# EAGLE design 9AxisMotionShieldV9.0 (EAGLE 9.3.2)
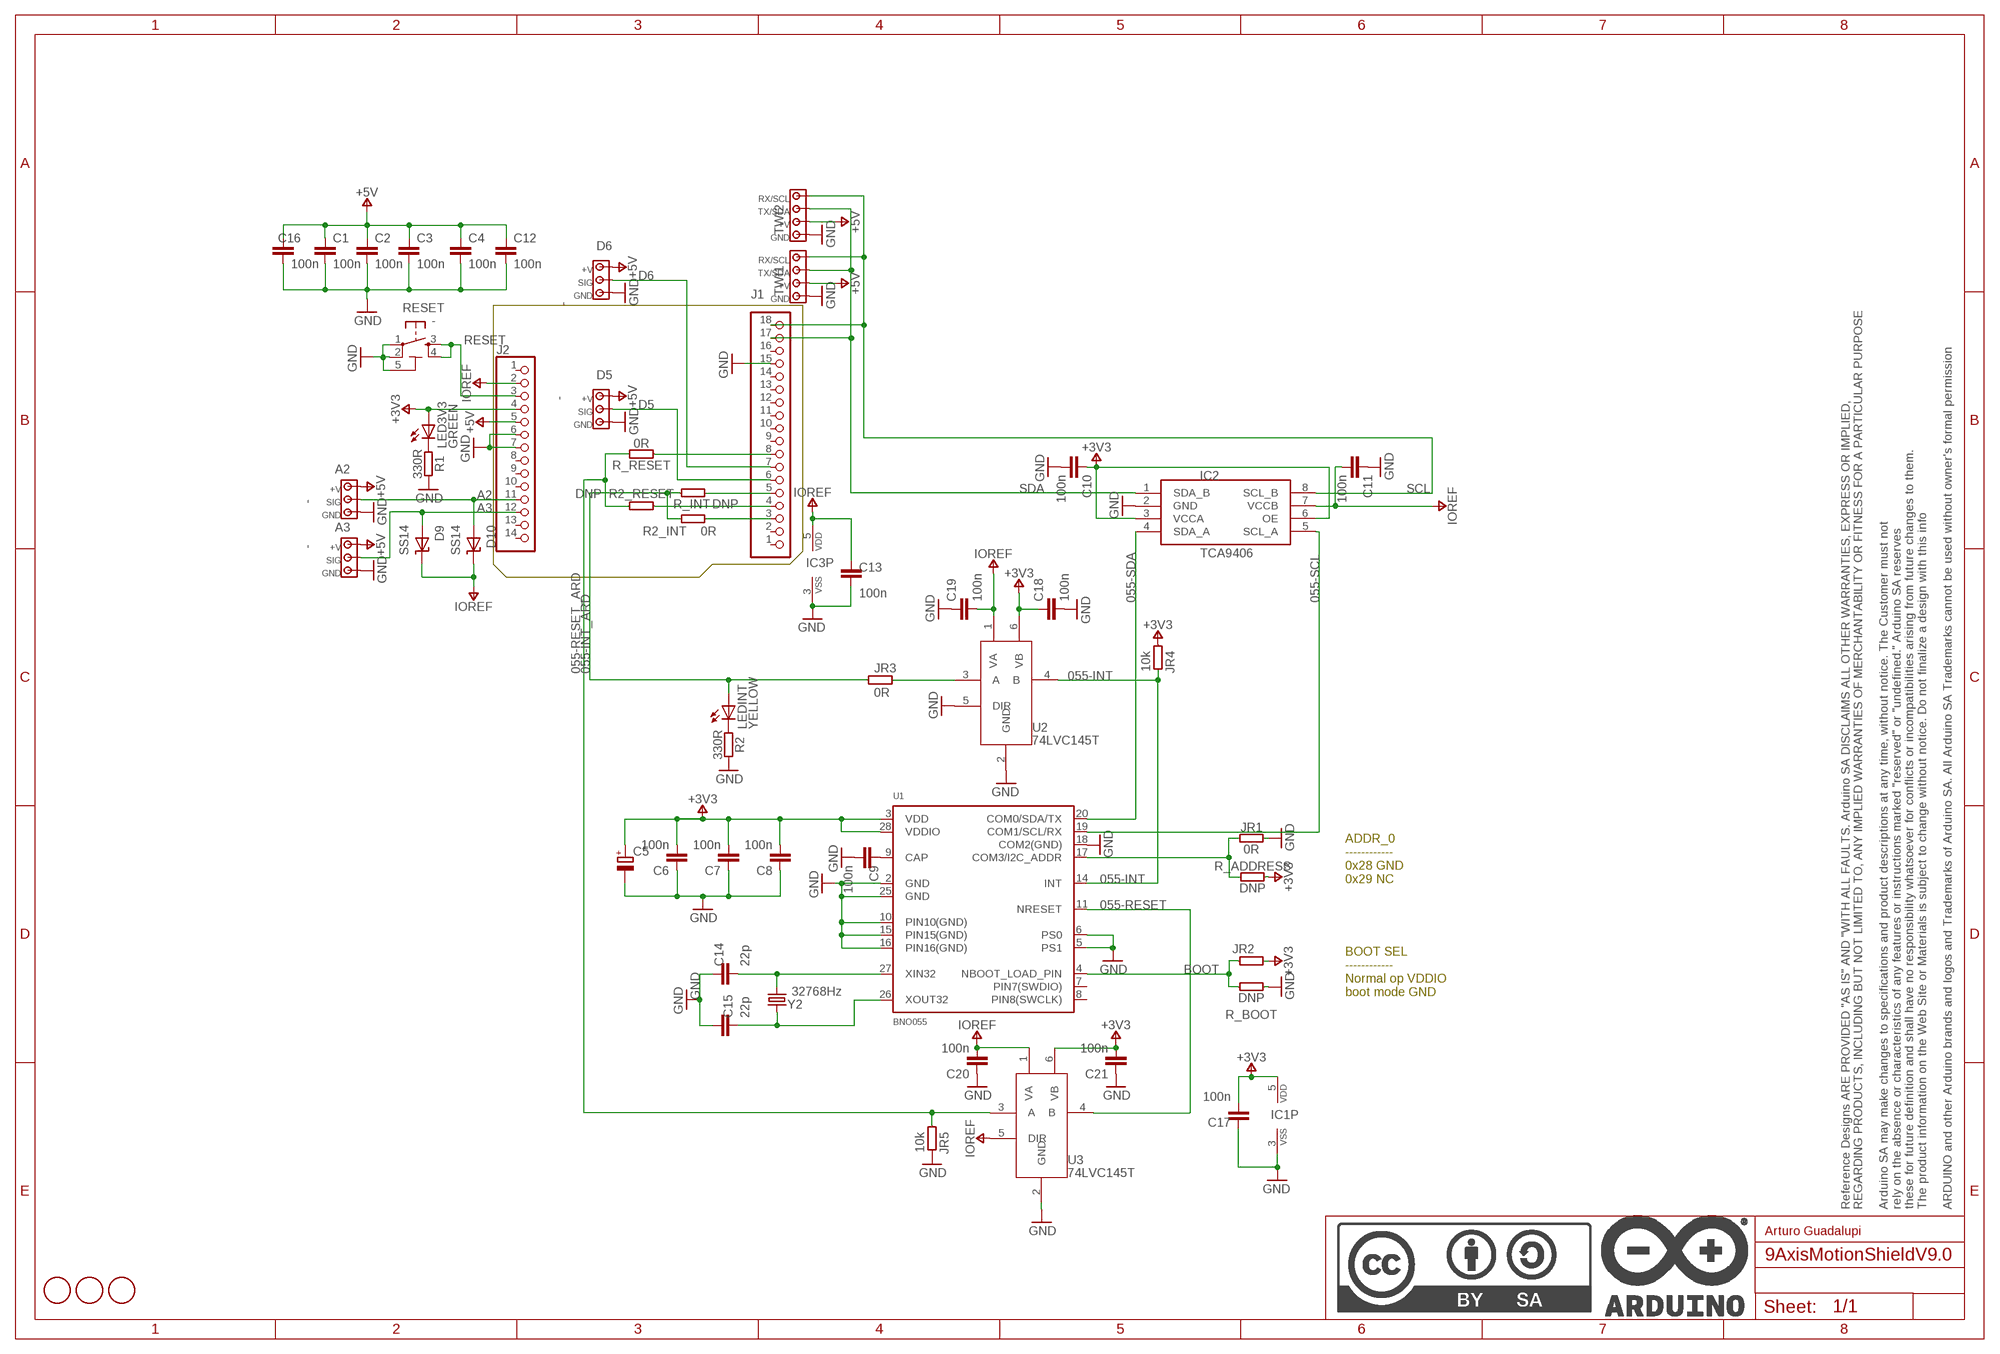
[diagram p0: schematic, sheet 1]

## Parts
A2  -  MODULINO-3  [MODULINO-3]
A3  -  MODULINO-3  [MODULINO-3]
C1  100n  C-100NF-0603  [0603-1608X90N]
C2  100n  C-100NF-0603  [0603-1608X90N]
C3  100n  C-100NF-0603  [0603-1608X90N]
C4  100n  C-100NF-0603  [0603-1608X90N]
C5  22u  0167_  [SMC_B]
C6  100n  C-100NF-0603  [0603-1608X90N]
C7  100n  C-100NF-0603  [0603-1608X90N]
C8  100n  C-100NF-0603  [0603-1608X90N]
C9  100n  C-100NF-0603  [0603-1608X90N]
C10  100n  C-100NF-0603  [0603-1608X90N]
C11  100n  C-100NF-0603  [0603-1608X90N]
C12  100n  C-100NF-0603  [0603-1608X90N]
C13  100n  C-100NF-0603  [0603-1608X90N]
C14  22p  C-22PF-0603  [0603-1608X90N]
C15  22p  C-22PF-0603  [0603-1608X90N]
C16  100n  C-100NF-0603  [0603-1608X90N]
C17  100n  C-100NF-0603  [0603-1608X90N]
C18  100n  C-100NF-0603  [0603-1608X90N]
C19  100n  C-100NF-0603  [0603-1608X90N]
C20  100n  C-100NF-0603  [0603-1608X90N]
C21  100n  C-100NF-0603  [0603-1608X90N]
D5  -  MODULINO-3  [MODULINO-3]
D6  -  MODULINO-3  [MODULINO-3]
D9  SS14  [SMA]
D10  SS14  [SMA]
FID1  DNP  FIDUCIAL-1.5MM  [FD-1-1.5]
FID2  DNP  FIDUCIAL-1.5MM  [FD-1-1.5]
FID3  DNP  FIDUCIAL-1.5MM  [FD-1-1.5]
FRAME1  DNP  A3-FRAME  [FRAME]
IC1  74LVC1G125DCKR  SN74LVC1G125DCKR  [SC70-5]
IC2  TCA9406  [SM-8]
IC3  74LVC1G125DCKR  SN74LVC1G125DCKR  [SC70-5]
J1  PINHD-1X18-SHIELD-CUSTOM  [1X18_]
J2  PINHD-1X14-MALE/FEMALE-CUSTOM  [1X14_]
JR1  0R  R-0R-0402  [0402-1005X55N]
JR2  0R  R-0R-0402  [0402-1005X55N]
JR3  0R  R-0R-0402  [0402-1005X55N]
JR4  10k  R-100K-0603  [C0603]
JR5  10k  R-100K-0603  [C0603]
LED3V3  GREEN  LED-GREEN-0805  [CHIPLED_0805]
LEDINT  YELLOW  LED-YELLOW-0805  [CHIPLED_0805]
R1  330R  R-330R-0402  [0402-1005X55N]
R2  330R  R-330R-0402  [0402-1005X55N]
R2_INT  0R  R-0R-0402  [0402-1005X55N]
R2_RESET  DNP  R-DNP-0402  [0402-1005X55N]
R_ADDRESS  DNP  R-DNP-0402  [0402-1005X55N]
R_BOOT  DNP  R-DNP-0402  [0402-1005X55N]
R_INT  DNP  R-DNP-0402  [0402-1005X55N]
R_RESET  0R  R-0R-0402  [0402-1005X55N]
RESET  -  TACTILE2  [TS42]
TWI1  TWI  MODULINO-4  [MODULINO-4]
TWI2  TWI  MODULINO-4  [MODULINO-4]
U1  BNO055  [BNO055]
U2  74LVC145T  SN74LVC1T45  [DCK]
U3  74LVC145T  SN74LVC1T45  [DCK]
Y2  32768Hz  32.768KHZ  [ABS07]

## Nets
055-INT: JR4.2 U1.14(INT) U2.4(B)
055-INT_ARD: JR3.1 LEDINT.A R2_INT.1 R_INT.1
055-RESET: U1.11(NRESET) U3.4(B)
055-RESET_ARD: JR5.1 R2_RESET.2 R_RESET.2 U3.3(A)
055-SCL: IC2.5(SCL_A) U1.19(COM1/SCL/RX)
055-SDA: IC2.4(SDA_A) U1.20(COM0/SDA/TX)
+3V3 [power]: C5.+ C6.2 C7.2 C8.2 C10.1 C17.2 C18.1 C21.2 IC1.5(VDD) IC2.3(VCCA) IC2.6(OE) J2.4 JR2.2 JR4.1 LED3V3.A R_ADDRESS.2 U1.3(VDD) U1.28(VDDIO) U2.6(VB) U3.6(VB)
+5V [power]: A2.1 A3.1 C1.1 C2.1 C3.1 C4.1 C12.1 C16.1 D5.1 D6.1 J2.5 TWI1.3 TWI2.3
A2: A2.2 D10.P$2(A) J2.11
A3: A3.2 D9.P$2(A) J2.12
ADDR_0: JR1.1 R_ADDRESS.1 U1.17(COM3/I2C_ADDR)
BOOT: JR2.1 R_BOOT.1 U1.4(NBOOT_LOAD_PIN)
D5: D5.2 J1.6
D6: D6.2 J1.7
GND [power]: A2.3 A3.3 C1.2 C2.2 C3.2 C4.2 C5.- C6.1 C7.1 C8.1 C9.2 C10.2 C11.1 C12.2 C13.2 C14.1 C15.1 C16.2 C17.1 C18.2 C19.1 C20.1 C21.1 D5.3 D6.3 IC1.3(VSS) IC2.2(GND) IC3.3(VSS) J1.15 J2.6 J2.7 JR1.2 JR5.2 R1.2 R2.2 R_BOOT.2 RESET.1 RESET.2 RESET.5(5-GND) TWI1.4 TWI2.4 U1.2(GND) U1.5(PS1) U1.6(PS0) U1.10(PIN10(GND)) U1.15(PIN15(GND)) U1.16(PIN16(GND)) U1.18(COM2(GND)) U1.25(GND) U2.2(GND) U2.5(DIR) U3.2(GND)
IOREF: C11.2 C13.1 C19.2 C20.2 D9.P$1(K) D10.P$1(K) IC2.7(VCCB) IC3.5(VDD) J2.2 U2.1(VA) U3.1(VA) U3.5(DIR)
N$1: LED3V3.C R1.1
N$3: C9.1 U1.9(CAP)
N$4: LEDINT.C R2.1
N$7: JR3.2 U2.3(A)
N$8: J1.3 R2_INT.2
N$10: J1.5 R_INT.2
N$11: J1.4 R2_RESET.1
N$56: J1.8 R_RESET.1
RESET: J2.3 RESET.3 RESET.4
SCL: IC2.8(SCL_B) J1.18 TWI1.1 TWI2.1
SDA: IC2.1(SDA_B) J1.17 TWI1.2 TWI2.2
XTAL1: C15.2 U1.26(XOUT32) Y2.1
XTAL2: C14.2 U1.27(XIN32) Y2.2
Unconnected: IC1.1(OE) IC1.2(I) IC1.4(O) IC3.1(OE) IC3.2(I) IC3.4(O) J1.1 J1.2 J1.9 J1.10 J1.11 J1.12 J1.13 J1.14 J1.16 J2.1 J2.8 J2.9 J2.10 J2.13 J2.14 U1.7(PIN7(SWDIO)) U1.8(PIN8(SWCLK))

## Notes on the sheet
- ADDR_0
  ------------
  0x28 GND
  0x29 NC
- BOOT SEL
  ------------
  Normal op VDDIO
  boot mode GND
- Arturo Guadalupi

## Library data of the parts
A2 A3 D5 D6 = Arduino-connectors:MODULINO-3: Polarized lock header 2.54mm pitch; CODE-ARDUINO: A5004; DATASHEET: https://www.alliedelec.com/m/d/412bc68f123f3befd9509afa982df40c.pdf; DISTRIBUTOR-LINK: https://www.alliedelec.com/adam-tech-lha-03-ts/70949176/; DISTRIBUTOR-PN: 70949176; MANUFACTURER: Adam Tech; MANUFACTURER-PN: LHA-03-TS
C1-C4 C6-C13 C16-C21 = Arduino-rcl:C: SMD Capacitor; CODE-ARDUINO: 0015; DATASHEET: http://search.murata.co.jp/Ceramy/image/img/A01X/G101/ENG/GRM188R71C104KA01-01.pdf; DISTRIBUTOR-LINK: https://www.digikey.com/product-detail/en/murata-electronics-north-america/GRM188R71C104KA01D/490-1532-1-ND/587771; DISTRIBUTOR-PN: 490-1532-2-ND; MANUFACTURER: Murata; MANUFACTURER-PN: GRM188R71C104KA01D; NOTE: -; PN-ALTERNATIVE1: NMC0603Y5V104Z25TRPF; PN-ALTERNATIVE2: C1608F104Z500NT; PN-ALTERNATIVE3: C0603C104K3RAC7411; PN-ALTERNATIVE4: 06035D104KAT2A; PN-ALTERNATIVE5: 0603B104K500CT
C5 = Condensatori:0167_: 22uF 25V; MONTHLY_USAGE: _____; PRICE: _____; SUPPLIER: _____; TYPE: Condensatori; VALUE: 22uF
C14 C15 = Arduino-rcl:C: SMD Capacitor; CODE-ARDUINO: 0014; DATASHEET: http://www.samsungsem.com/kr/support/product-search/mlcc/__icsFiles/afieldfile/2016/08/18/S_CL10C220JB8NNNC.pdf; DISTRIBUTOR-LINK: https://www.digikey.com/product-detail/en/samsung-electro-mechanics-america-inc/CL10C220JB8NNNC/1276-1023-1-ND/3889109; DISTRIBUTOR-PN: 1276-1023-1-ND; MANUFACTURER: Samsung; MANUFACTURER-PN: CL10C220JB8NNNC; NOTE: -; PN-ALTERNATIVE1: 0603N220J500CT
D9 D10 = SmartPrj:SS14: DIODE SS14 Diode Schottky 1A 40v
FID1-FID3 = Arduino-utility:FIDUCIAL: Fiducial mount; CODE-ARDUINO: DNP; DATASHEET: DNP; DISTRIBUTOR-LINK: DNP; DISTRIBUTOR-PN: DNP; MANUFACTURER: DNP; MANUFACTURER-PN: DNP
FRAME1 = Arduino-utility:A3-FRAME; CODE-ARDUINO: DNP; DATASHEET: DNP; DISTRIBUTOR-LINK: DNP; DISTRIBUTOR-PN: DNP; MANUFACTURER: DNP; MANUFACTURER-PN: DNP; NOTE: DNP
IC1 IC3 = Arduino-ICs:SN74LVC1G125DCKR: Single bus buffer with 3-state output; CODE-ARDUINO: 0040; DATASHEET: http://www.ti.com/lit/ds/symlink/sn74lvc1g125.pdf; DISTRIBUTOR-LINK: https://www.digikey.com/product-detail/en/texas-instruments/SN74LVC1G125DCKR/296-11604-1-ND/385743; DISTRIBUTOR-PN: 296-11604-1-ND; MANUFACTURER: Texas Instruments; MANUFACTURER-PN: SN74LVC1G125DCKR; NOTE: NO
IC2 = Arduino-ICs:TCA9406: I2C bidirectional level shifter; CODE-ARDUINO: A5381; DATASHEET: http://www.ti.com/lit/ds/symlink/tca9406.pdf; DISTRIBUTOR-LINK: https://www.digikey.com/product-detail/en/texas-instruments/TCA9406DCUR/296-28109-2-ND/2510728; DISTRIBUTOR-PN: 296-28109-2-ND; MANUFACTURER: TI; MANUFACTURER-PN: TCA9406DCUR
J1 = Arduino-connectors:PINHD-1X18: Pin header; CODE-ARDUINO: 3712
J2 = Arduino-connectors:PINHD-1X14: PIN HEADER; CODE-ARDUINO: 3711
JR1-JR3 R2_INT R_RESET = Arduino-rcl:R: SMD Resistor; CODE-ARDUINO: 0039; DATASHEET: www.yageo.com.tw/exep/pages/download/literatures/PYu-R_INT-thick_7.pdf; DISTRIBUTOR-LINK: http://www.digikey.com/product-detail/en/yageo/RC0402FR-070RL/311-0.0LRCT-ND/2827888; DISTRIBUTOR-PN: 311-0.0LRCT-ND; MANUFACTURER: Yageo; MANUFACTURER-PN: RC0402FR-070RL; NOTE: NO
JR4 JR5 = Arduino-rcl:R: SMD Resistor; CODE-ARDUINO: 0026; DATASHEET: http://www.yageo.com/documents/recent/PYu-RC_Group_51_RoHS_L_8.pdf; DISTRIBUTOR-LINK: https://www.digikey.com/product-detail/en/yageo/RC0603FR-07100KL/311-100KHRCT-ND/729836; DISTRIBUTOR-PN: 311-100KHRCT-ND; MANUFACTURER: Yageo; MANUFACTURER-PN: RC0603FR-07100KL; NOTE: NO
LED3V3 = Arduino-diodes:LED: LED; CODE-ARDUINO: 0043; DATASHEET: https://media.digikey.com/pdf/Data%20Sheets/Lite-On%20PDFs/LTST-C170GKT.pdf; DISTRIBUTOR-LINK: https://www.digikey.com/product-detail/it/lite-on-inc/LTST-C170GKT/160-1179-1-ND/269251; DISTRIBUTOR-PN: 160-1179-1-ND; MANUFACTURER: Lite-On; MANUFACTURER-PN: LTST-C170GKT; PN-ALTERNATIVE1: KPT-2012SGC
LEDINT = Arduino-diodes:LED: LED; CODE-ARDUINO: 0044; DATASHEET: https://media.digikey.com/pdf/Data%20Sheets/Lite-On%20PDFs/LTST-C170GKT.pdf; DISTRIBUTOR-LINK: https://www.digikey.com/product-detail/it/lite-on-inc/LTST-C170YKT/160-1175-1-ND/269247; DISTRIBUTOR-PN: 160-1175-1-ND; MANUFACTURER: Lite-On; MANUFACTURER-PN: LTST-C170YKT; PN-ALTERNATIVE1: KPT-2012YC
R1 R2 = Arduino-rcl:R: SMD Resistor; CODE-ARDUINO: 2229; DATASHEET: www.yageo.com.tw/exep/pages/download/literatures/PYu-R_INT-thick_7.pdf; DISTRIBUTOR-LINK: http://www.digikey.com/product-detail/en/yageo/RC0402FR-07330RL/311-330LRCT-ND/729541; DISTRIBUTOR-PN: 311-330LRCT-ND; MANUFACTURER: Yageo; MANUFACTURER-PN: RC0402FR-07330RL; NOTE: NO
R2_RESET R_ADDRESS R_BOOT R_INT = Arduino-rcl:R: SMD Resistor; CODE-ARDUINO: DNP; DATASHEET: DNP; DISTRIBUTOR-LINK: DNP; DISTRIBUTOR-PN: DNP; MANUFACTURER: DNP; MANUFACTURER-PN: DNP; NOTE: NO
RESET = Arduino-pushbuttons:TACTILE2: Pushbutton; CODE-ARDUINO: 0946; DATASHEET: http://www.mouser.com/ds/2/418/NG_CD_1571636_C1-122399.pdf; DISTRIBUTOR-LINK: https://www.mouser.it/ProductDetail/TE-Connectivity/1571636-3/?qs=%2fha2pyFaduiys%2fNUBzym%252bcoSb9tuK3Sjuv54qjf0hQ0%3d; DISTRIBUTOR-PN: 506-1571636-3; MANUFACTURER: TE; MANUFACTURER-PN: 1571636-3; PN-ALTERNATIVE1: TS42031-160WWS027260
TWI1 TWI2 = Arduino-connectors:MODULINO-4: Modulino 4 connector; CODE-ARDUINO: A5005; DATASHEET: https://www.tme.eu/en/Document/21cd81e6196d70241c99017ffcf9ebee/LHA-XX-TS.pdf; DISTRIBUTOR-LINK: https://www.tme.eu/en/details/lha-04-ts/raster-signal-connectors-254mm/adam-tech/; DISTRIBUTOR-PN: LHA-04-TS; MANUFACTURER: ADAM TECH; MANUFACTURER-PN: LHA-04-TS
U1 = Arduino-Sensors:BNO055: BNO055 - Motion Co-Processor; CODE-ARDUINO: 1658; DATASHEET: https://ae-bst.resource.bosch.com/media/_tech/media/datasheets/BST_BNO055_DS000_14.pdf; DISTRIBUTOR-LINK: http://www.digikey.com/product-detail/it/bosch-sensortec/BNO055/828-1058-1-ND/6136309; DISTRIBUTOR-PN: 828-1058-1-ND; MANUFACTURER: Bosch Sensortec; MANUFACTURER-PN: BNO055
U2 U3 = Arduino-ICs:SN74LVC1T45: SINGLE-BIT DUAL-SUPPLY BUS TRANSCEIVER WITH CONFIGURABLE VOLTAGE TRANSLATION AND 3-STATE OUTPUTS DIR = L B to A DIR = H (VVCA) A to B; CODE-ARDUINO: A5331; DATASHEET: http://www.ti.com/lit/ds/symlink/sn74lvc1t45-ep.pdf; DISTRIBUTOR-LINK: https://www.digikey.com/product-detail/en/texas-instruments/SN74LVC1T45DCKR/296-16844-1-ND/639460; DISTRIBUTOR-PN: 296-16844-1-ND; MANUFACTURER: TI; MANUFACTURER-PN: SN74LVC1T45DCKR; NOTE: NO
Y2 = Arduino-crystals:32.768KHZ: LF crystal; CODE-ARDUINO: 0213; DATASHEET: http://www.abracon.com/Resonators/ABS07.pdf; DISTRIBUTOR-LINK: http://www.digikey.com/product-detail/en/abracon-llc/ABS07-32.768KHZ-T/535-9542-1-ND/1237009; DISTRIBUTOR-PN: 535-9542-1-ND; MANUFACTURER: Abracon LLC; MANUFACTURER-PN: ABS07-32.768KHZ-T

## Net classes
1 power: width 0.254 mm, drill 0.3 mm, clearance 0.203 mm

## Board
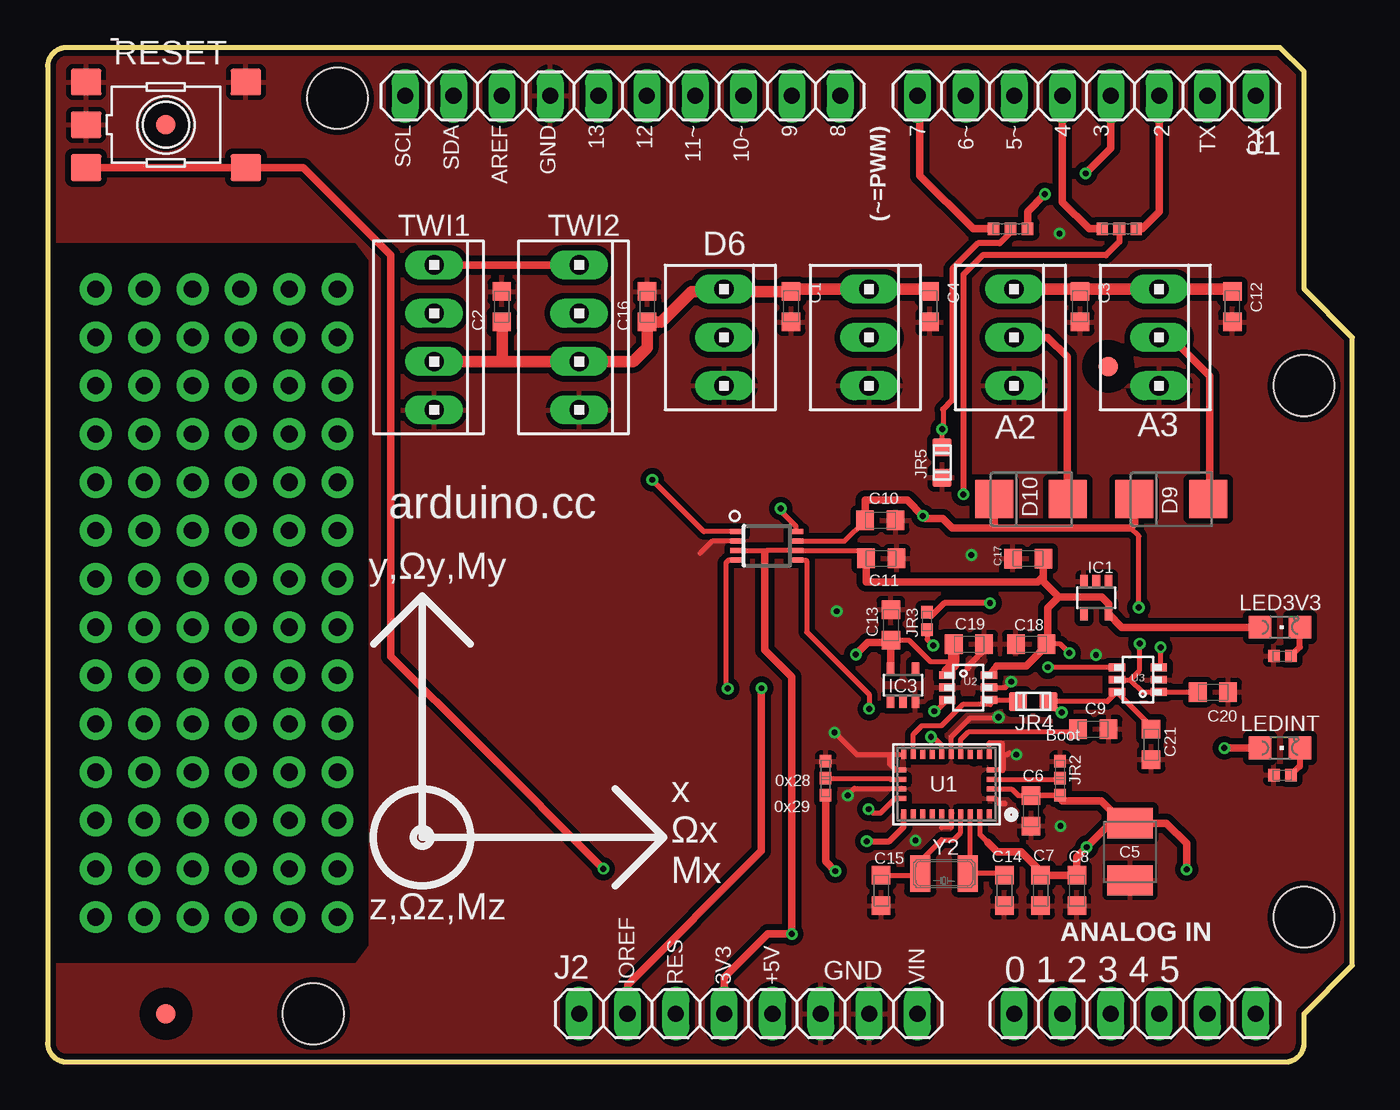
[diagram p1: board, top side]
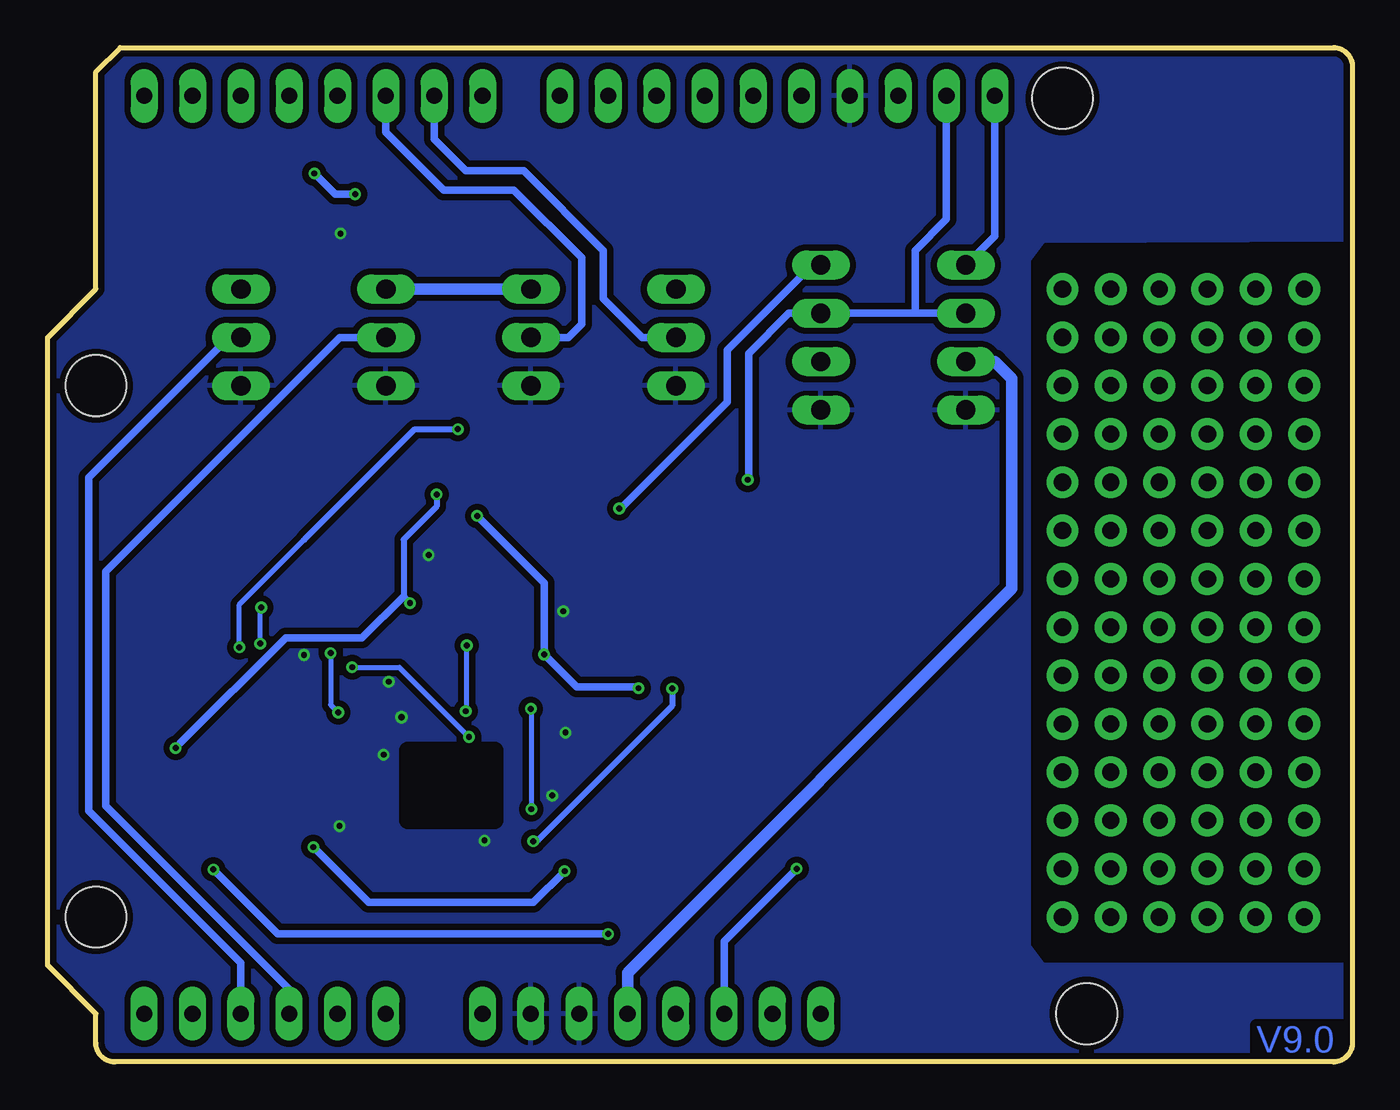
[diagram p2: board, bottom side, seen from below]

Size 68.58 x 53.34 mm. Coordinates in mm from the lower left corner, seen from the top.
Outline: 66.04,2.54 68.58,5.08 68.58,38.1 66.04,40.64 66.04,52.07 64.77,53.34 1,53.34 arc90 0,52.34 0,1 arc90 1,0 65.04,0 arc90 66.04,1 66.04,2.54
Copper layers (1*16): Top 0.035mm / dielectric 1.5mm / Bottom 0.035mm
Design rules "SeeedStudio_2layers *": minimum track width 6mil, minimum drill 0.3mm, track to track 6mil, track to pad 6mil, pad to pad 6mil, via to via 6mil, smd to smd 0mil, copper to edge 10mil, drill to drill 10mil, minimum pad ring 10mil, minimum via ring 6mil, stop-mask expansion 2mil, vias tented up to drill 100mil, thermal gap 10mil
Holes 3.2 mm at 66.04,35.56 66.04,7.62 15.24,50.67 13.97,2.54
tRestrict: 3 lines
bRestrict: 4 lines

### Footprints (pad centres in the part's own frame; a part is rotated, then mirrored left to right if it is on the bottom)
MODULINO-3 = drill 1.016 long: 1 -2.54,0; 2 0,0; 3 2.54,0
0603-1608X90N = smd 0.95 x 1: 1 -0.8,0; 2 0.8,0
SMC_B = smd 1.6 x 2.4: + -1.5,0; - 1.5,0
SMA = smd 2 x 2: P$1 -1.94,0; P$2 1.94,0
FD-1-1.5 = smd 1.016 x 1.016: P$1 0,0
SC70-5 = smd 0.4 x 0.7: 1 -0.65,-0.85; 2 0,-0.85; 3 0.65,-0.85; 4 0.65,0.85; 5 -0.65,0.85
SM-8 = smd 0.25 x 0.75: 1 -0.75,-1.55; 2 -0.25,-1.55; 3 0.25,-1.55; 4 0.75,-1.55; 5 0.75,1.55; 6 0.25,1.55; 7 -0.25,1.55; 8 -0.75,1.55
1X18_ = drill 0.85 pad 1.422 long: 1 -17.78,0; 2 -15.24,0; 3 -12.7,0; 4 -10.16,0; 5 -7.62,0; 6 -5.08,0; 7 -2.54,0; 8 0,0; 9 4.064,0; 10 6.604,0; 11 9.144,0; 12 11.684,0; 13 14.224,0; 14 16.764,0; 15 19.304,0; 16 21.844,0; 17 24.384,0; 18 26.924,0
1X14_ = drill 0.85 pad 1.422 long: 1 -17.78,0; 2 -15.24,0; 3 -12.7,0; 4 -10.16,0; 5 -7.62,0; 6 -5.08,0; 7 -2.54,0; 8 0,0; 9 5.08,0; 10 7.62,0; 11 10.16,0; 12 12.7,0; 13 15.24,0; 14 17.78,0
0402-1005X55N = smd 0.62 x 0.62: 1 -0.45,0; 2 0.45,0
C0603 = smd 0.95 x 1: 1 -0.8,0; 2 0.8,0
CHIPLED_0805 = smd 1.2 x 1.2: A -1.05,0; C 1.05,0
TS42 = smd 1.6 x 1.4: 1 4.2,-2.25; 2 -4.2,-2.25; 3 4.2,2.25; 4 -4.2,2.25; 5 4.2,0
MODULINO-4 = drill 1.016 long: 1 3.81,0; 2 1.27,0; 3 -1.27,0; 4 -3.81,0
BNO055 = smd 0.25 x 0.475: 1 -2.25,1.562; 6 -2.25,-1.562; 7 -1.75,-1.562; 8 -1.25,-1.562; 9 -0.75,-1.562; 10 -0.25,-1.562; 11 0.25,-1.562; 12 0.75,-1.562; 13 1.25,-1.562; 14 1.75,-1.562; 15 2.25,-1.562; 20 2.25,1.562; 21 1.75,1.562; 22 1.25,1.562; 23 0.75,1.562; 24 0.25,1.562; 25 -0.25,1.562; 26 -0.75,1.562; 27 -1.25,1.562; 28 -1.75,1.562 | smd 0.375 x 0.25: 2 -2.312,0.75; 3 -2.312,0.25; 4 -2.312,-0.25; 5 -2.312,-0.75; 16 2.312,-0.75; 17 2.312,-0.25; 18 2.312,0.25; 19 2.312,0.75
DCK = smd 0.9 x 0.4: 1 -1.1,0.65; 2 -1.1,0; 3 -1.1,-0.65; 4 1.1,-0.65; 5 1.1,0; 6 1.1,0.65
ABS07 = smd 1.1 x 1.9: 1 -1.25,0; 2 1.25,0

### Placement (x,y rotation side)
A2  50.8,38.1 270 top
A3  58.42,38.1 270 top
C1  39.08,39.71 270 top
C2  23.87,39.71 90 top
C3  54.27,39.71 270 top
C4  46.35,39.71 270 top
C5  56.9,11.05 270 top
C6  51.69,13.21 90 top
C7  52.2,9.02 90 top
C8  54.1,9.02 90 top
C9  54.97,17.5 0 top
C10  43.82,26.48 0 top
C11  43.77,28.48 180 top
C12  62.27,39.71 270 top
C13  44.32,22.99 90 top
C14  50.29,9.02 90 top
C15  43.81,9.02 90 top
C16  31.51,39.71 90 top
C17  51.54,26.47 0 top
C18  51.69,21.97 180 top
C19  48.43,21.97 180 top
C20  61.25,19.45 180 top
C21  58,16.7 90 top
D5  43.18,38.1 270 top
D6  35.56,38.1 270 top
D9  59.05,29.59 0 top
D10  51.69,29.59 0 top
FID1  6.22,49.28 180 top
FID2  6.22,2.54 0 top
FID3  55.75,36.58 0 top
FRAME1  0,0 0 top
IC1  55.12,24.41 180 top
IC2  37.8,27.14 270 top
IC3  44.96,19.81 0 top
J1  45.72,50.8 180 top
J2  45.72,2.54 0 top
JR1  40.89,15.37 90 top
JR2  53.21,14.48 270 top
JR3  46.22,23.19 270 top
JR4  51.8,18.95 180 top
JR5  47.02,31.52 270 top
LED3V3  64.77,22.86 0 top
LEDINT  64.77,16.51 0 top
R1  64.9,21.35 180 top
R2  64.9,15.08 180 top
R2_INT  56.77,43.81 0 top
R2_RESET  51.05,43.81 180 top
R_ADDRESS  40.89,14.48 270 top
R_BOOT  53.21,15.37 90 top
R_INT  55.88,43.81 180 top
R_RESET  50.16,43.81 0 top
RESET  6.22,49.28 180 top
TWI1  20.32,38.1 90 top
TWI2  27.94,38.1 90 top
U1  47.24,14.61 180 top
U2  48.39,19.68 0 top
U3  57.3,20.1 180 top
Y2  47.12,9.91 0 top

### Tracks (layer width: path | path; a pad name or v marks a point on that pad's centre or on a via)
055-INT
  Top 0.254: U1.14 45.49,17.22 45.95,17.68 46.98,17.68 48.1,18.8 49.55,18.8 U2.4 50.91,19.04 JR4.2
055-INT_ARD  (via drill 0.3)
  Top 0.254: JR3.1 46.42,23.44
  Top 0.305: R2_INT.1 R_INT.1 56.33,43.12 55.63,42.42 49.15,42.42 48.13,41.4 v48.13,29.84 | v49.53,24.13 47.12,24.13 46.42,23.44
  Top 0.406: v61.85,16.51 LEDINT.A
  Bottom 0.305: 61.59,16.76 v61.85,16.51 | v48.13,29.84 48.13,29.21 49.87,27.47 49.87,24.47 v49.53,24.13
  Bottom 0.406: 61.59,16.76 56.07,22.29 52.06,22.29 49.87,24.47
055-RESET  (via drill 0.3)
  Top 0.254: U1.11 46.99,16.64 46.54,17.09 v46.43,17.09 | U3.4 v52.57,20.75
  Bottom 0.254: v46.43,17.09 50.1,20.75 v52.57,20.75
055-RESET_ARD  (via drill 0.3)
  Top 0.254: U3.3 58.5,20.85 v58.5,21.8 | 47.07,34.31 47.07,33.33 v47.02,33.28 JR5.1
  Top 0.305: R_RESET.2 50.62,43.63 50.04,43.05 48.9,43.05 47.55,41.71 47.55,34.8 47.07,34.31
  Top 0.406: R_RESET.2 R2_RESET.2
  Bottom 0.254: v58.5,21.8 58.5,24.05 55.02,27.52
  Bottom 0.305: v47.02,33.28 49.27,33.28 55.02,27.52 55.12,27.43
055-SCL  (via drill 0.3)
  Top 0.254: v43.18,18.57 43.18,19.33 39.9,22.61 39.9,26.35 39.86,26.39 IC2.5 | v43.16,13.3 43.37,13.08 43.78,13.08 44.55,13.86 U1.19
  Bottom 0.254: v43.18,18.57 43.16,18.54 v43.16,13.3
055-SDA  (via drill 0.3)
  Top 0.254: U1.20 | IC2.4 35.79,26.39 35.65,26.25 35.65,19.73 v35.75,19.63
  Top 0.305: v43.05,11.61 44.25,11.61 44.99,12.35 U1.20
  Bottom 0.305: v35.75,19.63 35.75,18.73 42.88,11.61 v43.05,11.61
+3V3  (via drill 0.3)
  Top 0.254: JR2.2 53.33,13.92 53.33,13.72 | 56.64,12.65 56.44,12.65 | U1.3 50.67,14.36 51.02,14.01 51.27,14.01 C6.2 51.73,14.01 51.75,14.03 | U1.28 48.99,11.97 49.4,11.56 | C21.2 58,17.65 U3.6 55.7,18.95 JR4.1 53.17,18.38 v53.3,18.38 | v53.7,21.5 53.23,21.97 C18.1 | C10.1 42.61,26.89 IC2.6 37.77,26.89 | 37.77,26.89 37.69,26.82 | IC2.3 37.77,26.89
  Top 0.305: 51.75,14.03 JR2.2
  Top 0.406: 53.33,13.72 55.37,13.72 56.33,12.76 | 56.33,12.76 56.44,12.65 | 56.33,12.76 56.07,12.76 v54.61,11.3 54.1,10.79 C8.2 C7.2 52.2,10.03 51.18,11.05 49.91,11.05 49.4,11.56 | v41.4,10.03 40.89,10.54 R_ADDRESS.2 | C10.1 43.02,25.25 52.05,25.25 52.34,25.54 | 56.64,12.65 56.74,12.55 C5.+ 58.8,12.55 59.87,11.48 v59.87,10.12 | 52.34,25.54 C17.2 | U2.6 49.88,20.83 51.44,20.83 52.49,21.88 C18.1 52.66,22.14 52.58,22.23 52.58,23.88 53.15,24.45 | 52.34,25.54 52.34,25.26 53.15,24.45 | LED3V3.A 56.47,22.86 IC1.5 55.77,24.08 55.4,24.45 53.15,24.45 | 37.69,26.82 37.7,26.8 37.7,21.66 39.12,20.25 v39.12,6.73 37.85,6.73 35.56,4.45 J2.4
  Bottom 0.254: v53.7,21.5 53.7,18.78 v53.3,18.38
  Bottom 0.406: v41.4,10.03 43.05,8.38 51.69,8.38 v54.61,11.3 | v39.12,6.73 56.48,6.73 v59.87,10.12
+5V
  Top 0.305: D6.1 35.69,40.51
  Top 0.61: C4.1 46.23,40.64 D5.1 39.2,40.64 C1.1 35.69,40.51 33.86,40.51 32.26,38.91 C16.1 31.51,37.55 30.79,36.83 TWI2.3 23.9,36.83 | C3.1 54.39,40.64 | 54.39,40.64 A3.1 62.14,40.64 C12.1 | A2.1 54.39,40.64 | TWI1.3 23.9,36.83 | C2.1 23.9,38.88 23.9,36.83
  Bottom 0.61: TWI1.3 18.8,36.83 17.91,35.94 17.91,24.89 38.1,4.7 J2.5 | D5.1 A2.1
A2
  Top 0.406: D10.P$2 53.59,29.63 53.59,37.08 52.58,38.1 A2.2
  Bottom 0.406: J2.11 55.88,3.81 65.53,13.46 65.53,25.78 53.21,38.1 A2.2
A3
  Top 0.406: D9.P$2 61.09,29.68 61.09,36.07 59.05,38.1 A3.2
  Bottom 0.406: J2.12 58.42,5.21 66.42,13.21 66.42,30.73 59.05,38.1 A3.2
ADDR_0
  Top 0.254: U1.17 44.3,14.86 44.27,14.89 40.92,14.89 JR1.1 | R_ADDRESS.1 40.93,14.81
  Top 0.305: R_ADDRESS.1 JR1.1
BOOT
  Top 0.254: U1.4 53.15,14.86 R_BOOT.1
  Top 0.406: JR2.1 R_BOOT.1 53.15,14.86
D5
  Bottom 0.406: J1.6 50.8,48.9 47.75,45.85 44.07,45.85 40.51,42.29 40.51,38.79 41.2,38.1 D5.2
D6
  Bottom 0.406: J1.7 48.26,48.51 46.61,46.86 43.56,46.86 39.37,42.67 39.37,40.13 37.34,38.1 D6.2
GND  (via drill 0.3, 0.35)
  Top 0.254: 50.55,16.26 50.46,16.17 50.2,16.17 50.16,16.17 50.16,16.75 50.12,16.8 49.5,16.8 49.49,16.79 U1.6 | 50.2,15.36 U1.5 | 47.49,12.32 U1.25 47.54,13.09 | 47.49,12.32 47.5,12.32 | U1.18 44.89,14.4 42.41,14.4 42.05,14.04 v42.05,14.01 | v41.36,17.32 42.52,16.17 44.2,16.17 | 44.2,16.17 U1.15 | 44.2,16.17 44.26,16.1 44.26,15.67 44.58,15.36 U1.16 | 47.49,12.32 46.99,12.32 | U2.5 50.34,19.68 v50.65,20 | IC2.2 34.94,27.39 34.3,26.75 | U1.10 47.49,17.09 47.54,17.14 48.48,18.09 49.93,18.09 v49.97,18.13
  Top 0.305: U1.2 49.77,13.86 50.04,13.59 50.29,13.59 | 50.2,16.17 50.2,15.36 | C19.1 49.23,21.67 48.39,20.83 48.39,20.7
  Top 0.406: C13.2 44.48,24.03
  other vias: 53.24,12.41 41.48,23.7 48.55,26.66 53.19,43.56 45.62,11.65 50.92,16.16 55.1,21.4
  pour Bottom (isolate 0.33): 68.58,0 0,0 0,5.08 16.26,5.08 17.02,6.1 17.02,42.16 16.26,43.18 0,43.26 0,53.34 68.58,53.34
  pour Top (isolate 0.305): 68.58,53.34 68.58,0 0,0 0,5.08 16.26,5.08 17.02,6.1 17.02,42.16 16.26,43.18 0,43.18 0,53.34
IOREF  (via drill 0.3)
  Top 0.254: U3.5 56.9,20.1 | 56.9,20.1 57.55,19.45 U3.1 C20.2 | 56.9,20.1 57.4,20.6 v57.4,22 | v57.35,23.9 57.35,27.65 56.91,28.09 | C13.1 45.26,22.19 46.4,21.05 47.58,21.05 47.59,21.06 47.63,21.1 | 47.29,20.56 U2.1 | IC2.7 41.88,27.39 C11.2
  Top 0.305: IC3.5 44.32,21.06
  Top 0.405: v37.52,19.66 37.52,11.1 30.48,4.06 | v42.48,21.43 43.12,22.06 44.32,22.06 | 46.52,28.57 47.05,28.57
  Top 0.406: 44.32,21.06 44.32,22.06 C13.1 | 49.76,28.07 56.9,28.07 56.91,28.09 57.15,28.32 57.15,29.56 D9.P$1 | 49.76,28.07 49.75,28.08 D10.P$1 | 49.76,28.07 47.56,28.07 47.05,28.57 | C11.2 42.97,29.54 45.17,29.54 v46,28.71 46.14,28.57 46.52,28.57 | J2.2 30.48,4.06
  Top 0.61: 47.29,20.56 47.59,20.86 47.59,21.06 | C19.2 47.63,21.1
  Bottom 0.254: v57.4,22 57.4,23.85 v57.35,23.9
  Bottom 0.405: v37.52,19.66 37.57,19.71 40.77,19.71 v42.48,21.43 42.48,25.2 v46,28.71
N$1
  Top 0.305: R1.1 65.82,21.82 LED3V3.C
N$3
  Top 0.254: U1.9 47.99,16.95 48.4,17.36 54.02,17.36 C9.1
N$4
  Top 0.305: LEDINT.C 65.82,15.57 65.81,15.53 65.8,15.53 R2.1
N$6  (via drill 0.9 pad 1.68)
  other vias: 2.54,33.02
N$7  (via drill 0.3)
  Top 0.254: U2.3 46.7,18.45 v46.6,18.45 | JR3.2 46.22,22.23 v46.55,21.9
  Bottom 0.254: v46.6,18.45 46.55,18.5 v46.55,21.9
N$8
  Top 0.406: J1.3 58.42,44.7 57.53,43.81 R2_INT.2
N$10
  Top 0.406: J1.5 53.34,45.21 54.74,43.81 R_INT.2
N$11  (via drill 0.3)
  Top 0.406: v52.41,45.63 51.5,44.72 R2_RESET.1 | v54.56,46.72 55.88,48.04 J1.4
  Bottom 0.406: v54.56,46.72 53.47,45.63 v52.41,45.63
N$12  (via drill 0.9 pad 1.68)
  other vias: 5.08,33.02
N$13  (via drill 0.9 pad 1.68)
  other vias: 7.62,33.02
N$14  (via drill 0.9 pad 1.68)
  other vias: 10.16,33.02
N$15  (via drill 0.9 pad 1.68)
  other vias: 12.7,33.02
N$16  (via drill 0.9 pad 1.68)
  other vias: 2.54,25.4
N$17  (via drill 0.9 pad 1.68)
  other vias: 5.08,25.4
N$18  (via drill 0.9 pad 1.68)
  other vias: 7.62,25.4
N$19  (via drill 0.9 pad 1.68)
  other vias: 10.16,25.4
N$20  (via drill 0.9 pad 1.68)
  other vias: 12.7,25.4
N$21  (via drill 0.9 pad 1.68)
  other vias: 12.7,22.86
N$22  (via drill 0.9 pad 1.68)
  other vias: 10.16,22.86
N$23  (via drill 0.9 pad 1.68)
  other vias: 7.62,22.86
N$24  (via drill 0.9 pad 1.68)
  other vias: 5.08,22.86
N$25  (via drill 0.9 pad 1.68)
  other vias: 2.54,22.86
N$26  (via drill 0.9 pad 1.68)
  other vias: 2.54,20.32
N$27  (via drill 0.9 pad 1.68)
  other vias: 5.08,20.32
N$28  (via drill 0.9 pad 1.68)
  other vias: 7.62,20.32
N$29  (via drill 0.9 pad 1.68)
  other vias: 10.16,20.32
N$30  (via drill 0.9 pad 1.68)
  other vias: 12.7,20.32
N$31  (via drill 0.9 pad 1.68)
  other vias: 12.7,17.78
N$32  (via drill 0.9 pad 1.68)
  other vias: 10.16,17.78
N$33  (via drill 0.9 pad 1.68)
  other vias: 7.62,17.78
N$34  (via drill 0.9 pad 1.68)
  other vias: 5.08,17.78
N$35  (via drill 0.9 pad 1.68)
  other vias: 2.54,17.78
N$36  (via drill 0.9 pad 1.68)
  other vias: 2.54,15.24
N$37  (via drill 0.9 pad 1.68)
  other vias: 5.08,15.24
N$38  (via drill 0.9 pad 1.68)
  other vias: 7.62,15.24
N$39  (via drill 0.9 pad 1.68)
  other vias: 10.16,15.24
N$40  (via drill 0.9 pad 1.68)
  other vias: 12.7,15.24
N$41  (via drill 0.9 pad 1.68)
  other vias: 12.7,12.7
N$42  (via drill 0.9 pad 1.68)
  other vias: 10.16,12.7
N$43  (via drill 0.9 pad 1.68)
  other vias: 7.62,12.7
N$44  (via drill 0.9 pad 1.68)
  other vias: 5.08,12.7
N$45  (via drill 0.9 pad 1.68)
  other vias: 2.54,12.7
N$46  (via drill 0.9 pad 1.68)
  other vias: 2.54,10.16
N$47  (via drill 0.9 pad 1.68)
  other vias: 5.08,10.16
N$48  (via drill 0.9 pad 1.68)
  other vias: 7.62,10.16
N$49  (via drill 0.9 pad 1.68)
  other vias: 10.16,10.16
N$50  (via drill 0.9 pad 1.68)
  other vias: 12.7,10.16
N$51  (via drill 0.9 pad 1.68)
  other vias: 12.7,7.62
N$52  (via drill 0.9 pad 1.68)
  other vias: 10.16,7.62
N$53  (via drill 0.9 pad 1.68)
  other vias: 7.62,7.62
N$54  (via drill 0.9 pad 1.68)
  other vias: 5.08,7.62
N$55  (via drill 0.9 pad 1.68)
  other vias: 2.54,7.62
N$56
  Top 0.406: R_RESET.1 48.64,43.81 45.85,46.61 45.85,50.67 J1.8
N$62  (via drill 0.9 pad 1.68)
  other vias: 15.24,7.62
N$63  (via drill 0.9 pad 1.68)
  other vias: 15.24,10.16
N$64  (via drill 0.9 pad 1.68)
  other vias: 15.24,12.7
N$65  (via drill 0.9 pad 1.68)
  other vias: 15.24,15.24
N$66  (via drill 0.9 pad 1.68)
  other vias: 15.24,17.78
N$67  (via drill 0.9 pad 1.68)
  other vias: 15.24,20.32
N$68  (via drill 0.9 pad 1.68)
  other vias: 15.24,27.94
N$69  (via drill 0.9 pad 1.68)
  other vias: 15.24,25.4
N$70  (via drill 0.9 pad 1.68)
  other vias: 15.24,22.86
N$71  (via drill 0.9 pad 1.68)
  other vias: 15.24,30.48
N$72  (via drill 0.9 pad 1.68)
  other vias: 12.7,30.48
N$73  (via drill 0.9 pad 1.68)
  other vias: 10.16,30.48
N$74  (via drill 0.9 pad 1.68)
  other vias: 7.62,30.48
N$75  (via drill 0.9 pad 1.68)
  other vias: 5.08,30.48
N$76  (via drill 0.9 pad 1.68)
  other vias: 2.54,30.48
N$77  (via drill 0.9 pad 1.68)
  other vias: 2.54,27.94
N$78  (via drill 0.9 pad 1.68)
  other vias: 5.08,27.94
N$79  (via drill 0.9 pad 1.68)
  other vias: 7.62,27.94
N$80  (via drill 0.9 pad 1.68)
  other vias: 10.16,27.94
N$81  (via drill 0.9 pad 1.68)
  other vias: 12.7,27.94
N$82  (via drill 0.9 pad 1.68)
  other vias: 15.24,33.02
N$83  (via drill 0.9 pad 1.68)
  other vias: 15.24,35.56
N$84  (via drill 0.9 pad 1.68)
  other vias: 12.7,35.56
N$85  (via drill 0.9 pad 1.68)
  other vias: 10.16,35.56
N$86  (via drill 0.9 pad 1.68)
  other vias: 7.62,35.56
N$87  (via drill 0.9 pad 1.68)
  other vias: 5.08,35.56
N$88  (via drill 0.9 pad 1.68)
  other vias: 2.54,35.56
N$89  (via drill 0.9 pad 1.68)
  other vias: 2.54,38.1
N$90  (via drill 0.9 pad 1.68)
  other vias: 5.08,38.1
N$91  (via drill 0.9 pad 1.68)
  other vias: 7.62,38.1
N$92  (via drill 0.9 pad 1.68)
  other vias: 10.16,38.1
N$93  (via drill 0.9 pad 1.68)
  other vias: 12.7,38.1
N$94  (via drill 0.9 pad 1.68)
  other vias: 15.24,38.1
N$95  (via drill 0.9 pad 1.68)
  other vias: 15.24,40.64
N$96  (via drill 0.9 pad 1.68)
  other vias: 12.7,40.64
N$97  (via drill 0.9 pad 1.68)
  other vias: 10.16,40.64
N$98  (via drill 0.9 pad 1.68)
  other vias: 7.62,40.64
N$99  (via drill 0.9 pad 1.68)
  other vias: 5.08,40.64
N$100  (via drill 0.9 pad 1.68)
  other vias: 2.54,40.64
RESET  (via drill 0.3)
  Top 0.406: v29.21,10.16 22.68,16.69 18.03,21.34 18.03,42.42 13.43,47.03 RESET.4 RESET.3 3.56,47.03
  Bottom 0.406: v29.21,10.16 33.02,6.35 J2.3
SCL  (via drill 0.3)
  Top 0.254: IC2.8 39.35,28.16 38.54,28.98
  Top 0.305: 38.54,28.98 v38.54,29.1
  Top 0.406: TWI1.1 TWI2.1
  Bottom 0.405: 32.87,34.69 38.46,29.1 v38.54,29.1
  Bottom 0.406: TWI1.1 18.8,43.43 J1.18 | 32.87,34.69 32.87,37.44 28.39,41.91 TWI2.1
SDA  (via drill 0.3)
  Top 0.254: IC2.1 34.49,27.89 31.78,30.61 v31.78,30.62
  Bottom 0.305: v31.78,30.62 31.73,30.67
  Bottom 0.406: 31.73,30.67 31.73,37.26 29.62,39.37 TWI2.2 23.05,39.37 | J1.17 21.34,44.32 22.99,42.67 22.99,39.43 23.05,39.37 | 23.05,39.37 TWI1.2
XTAL1
  Top 0.254: C15.2 45.78,9.82 Y2.1 45.87,10.56 46.99,11.68 47.62,11.68 47.99,12.05 U1.26
XTAL2
  Top 0.254: U1.27 48.49,10.03 Y2.2 50.2,9.91 C14.2

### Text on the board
Bottom: V9.0
tPlace: y,Ωy,My | Boot | 0x28 | 0x29 | x / Ωx / Mx | z,Ωz,Mz
tNames: SCL | SDA | AREF | GND | 13 | 12 | 11~ | 10~ | 9 | 8 | 7 | 6~ | 5~ | 4 | 3 | 2 | TX | RX | (~=PWM) | arduino.cc | ANALOG IN | IOREF | RES | 3V3 | +5V | GND | VIN | 0 1 2 3 4 5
